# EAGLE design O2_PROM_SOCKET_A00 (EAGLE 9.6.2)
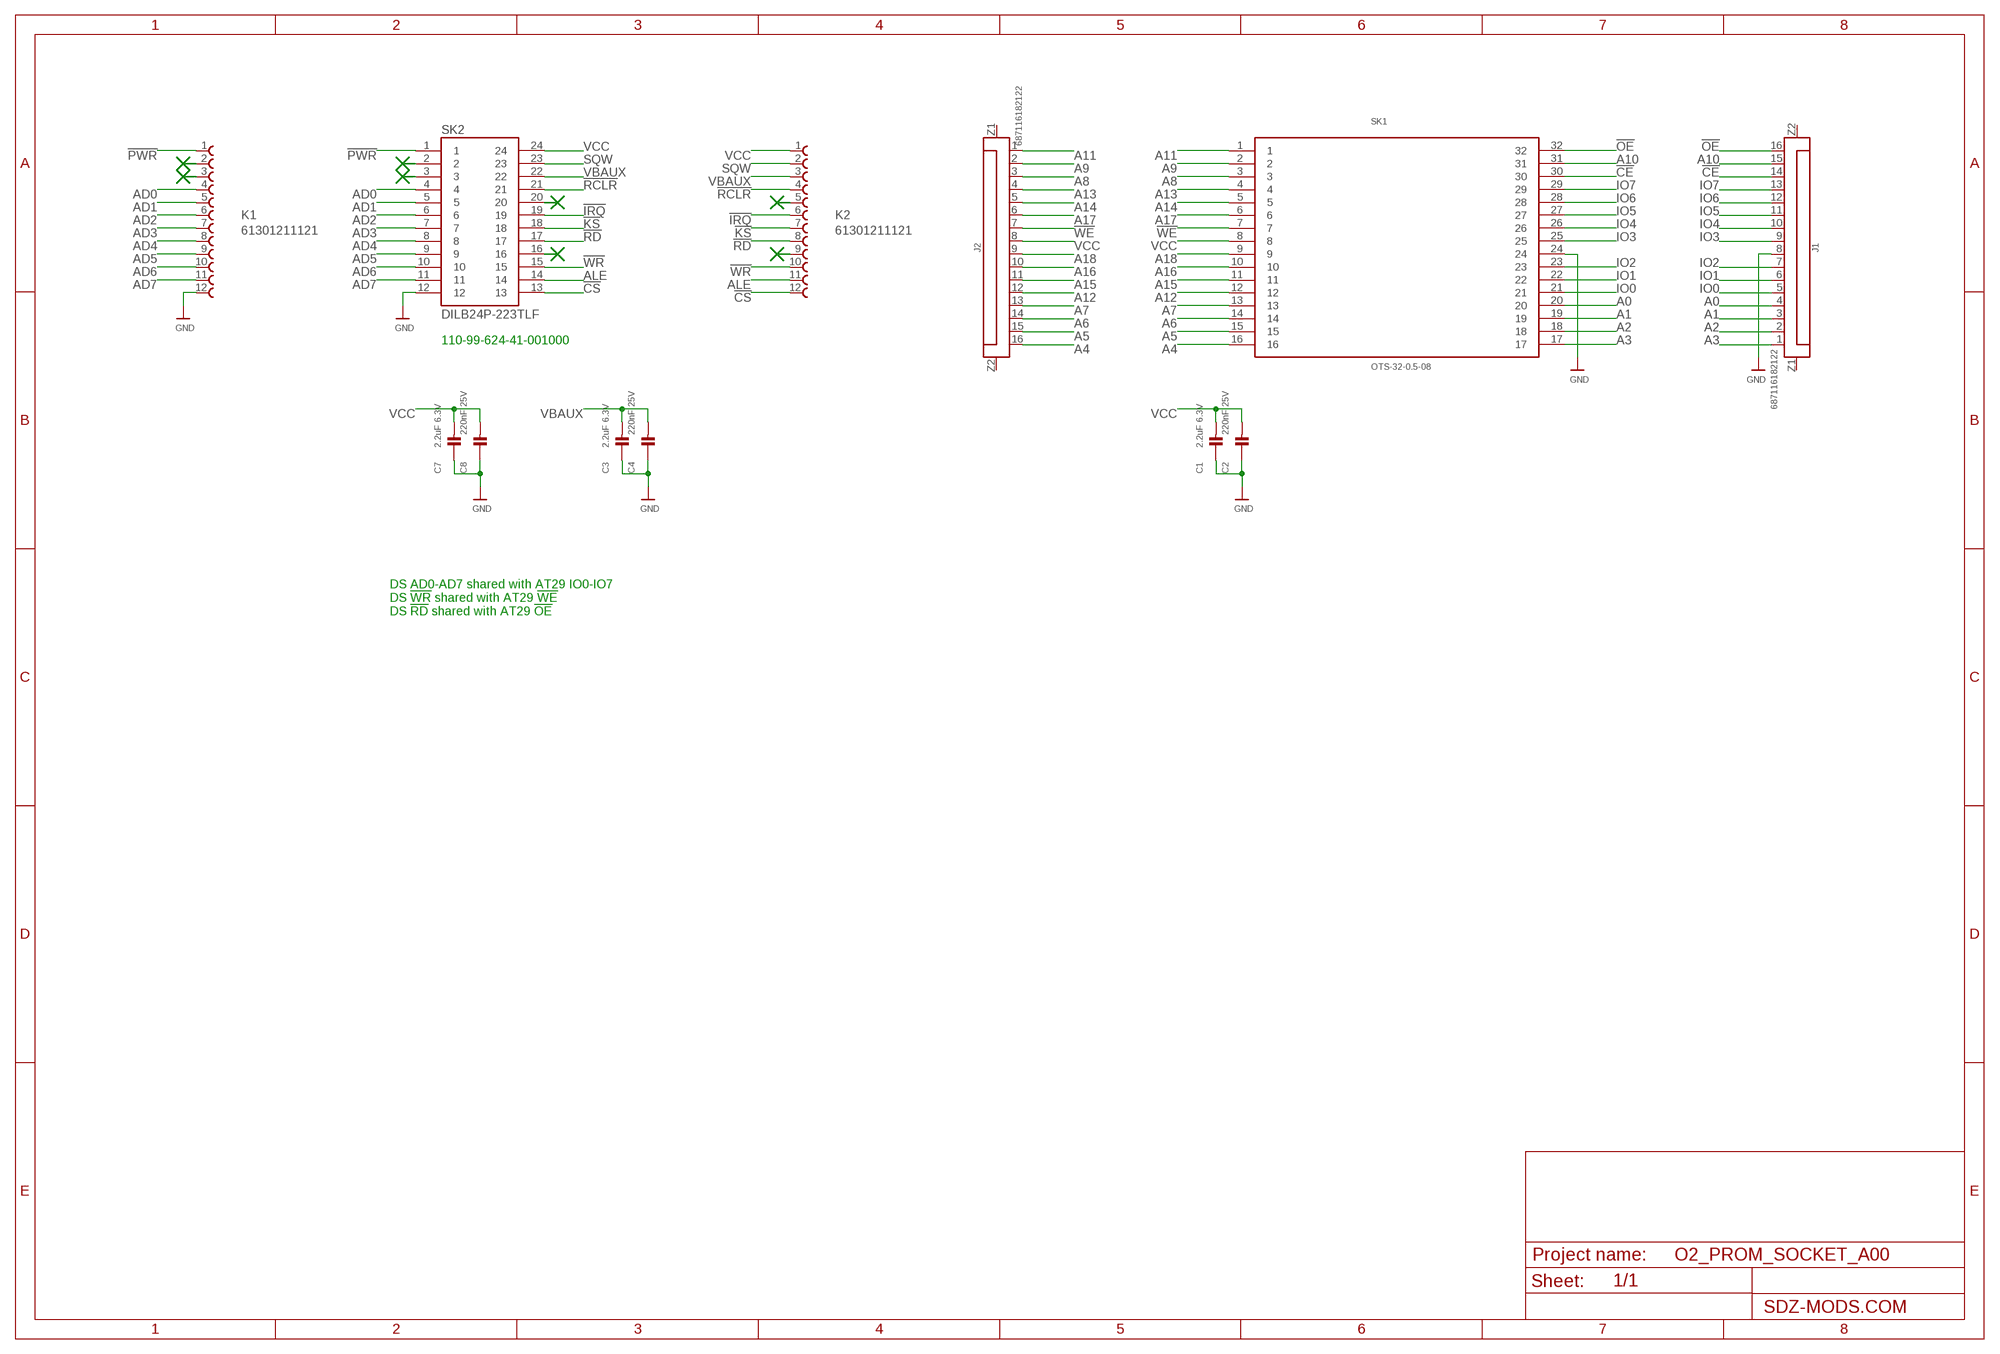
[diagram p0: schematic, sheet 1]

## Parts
C1  2.2uF 6.3V  CAP_CERAMIC0402D  [0402D]
C2  220nF 25V  CAP_CERAMIC0402D  [0402D]
C3  2.2uF 6.3V  CAP_CERAMIC0402D  [0402D]
C4  220nF 25V  CAP_CERAMIC0402D  [0402D]
C7  2.2uF 6.3V  CAP_CERAMIC0402D  [0402D]
C8  220nF 25V  CAP_CERAMIC0402D  [0402D]
J1  687116182122  6871XX182122_687116182122  [687116182122]
J2  687116182122  6871XX182122_687116182122  [687116182122]
K1  61301211121  [61301211121]
K2  61301211121  [61301211121]
SK1  OTS-32-0.5-08  [OTS-32-0.5-08]
SK2  DILB24P-223TLF  [AMPHENOL_DILB24P-223TLF]

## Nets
!CE: J1.14 SK1.30
!CS: K2.12 SK2.13
!IRQ: K2.6 SK2.19
!KS: K2.7 SK2.18
!OE: J1.16 SK1.32
!PWR: K1.1 SK2.1
!RCLR: K2.4 SK2.21
!RD: K2.8 SK2.17
!WE: J2.7 SK1.7
!WR: K2.10 SK2.15
A0: J1.4 SK1.20
A1: J1.3 SK1.19
A2: J1.2 SK1.18
A3: J1.1 SK1.17
A4: J2.16 SK1.16
A5: J2.15 SK1.15
A6: J2.14 SK1.14
A7: J2.13 SK1.13
A8: J2.3 SK1.3
A9: J2.2 SK1.2
A10: J1.15 SK1.31
A11: J2.1 SK1.1
A12: J2.12 SK1.12
A13: J2.4 SK1.4
A14: J2.5 SK1.5
A15: J2.11 SK1.11
A16: J2.10 SK1.10
A17: J2.6 SK1.6
A18: J2.9 SK1.9
AD0: K1.4 SK2.4
AD1: K1.5 SK2.5
AD2: K1.6 SK2.6
AD3: K1.7 SK2.7
AD4: K1.8 SK2.8
AD5: K1.9 SK2.9
AD6: K1.10 SK2.10
AD7: K1.11 SK2.11
ALE: K2.11 SK2.14
GND: C1.3 C2.3 C3.3 C4.3 C7.3 C8.3 J1.8 K1.12 SK1.24 SK2.12
IO0: J1.5 SK1.21
IO1: J1.6 SK1.22
IO2: J1.7 SK1.23
IO3: J1.9 SK1.25
IO4: J1.10 SK1.26
IO5: J1.11 SK1.27
IO6: J1.12 SK1.28
IO7: J1.13 SK1.29
SQW: K2.2 SK2.23
VBAUX: C3.4 C4.4 K2.3 SK2.22
VCC: C1.4 C2.4 C7.4 C8.4 J2.8 K2.1 SK1.8 SK2.24
Unconnected: J1.Z1 J1.Z2 J2.Z1 J2.Z2 K1.2 K1.3 K2.5 K2.9 SK2.2 SK2.3 SK2.16 SK2.20

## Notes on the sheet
- 110-99-624-41-001000
- DS AD0-AD7 shared with AT29 IO0-IO7
  DS !WR! shared with AT29 !WE!
  DS !RD! shared with AT29 !OE!

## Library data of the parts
C1-C4 C7 C8 = microbuilder:CAP_CERAMIC: Ceramic Capacitors
J1 J2 = Eagle_WR-FPC (rev24a):6871XX182122_687116182122: WR-FPC 0.50 mm SMT ZIF Horizontal Dual Contact KIND PROPERTIES Pitch 0.5 mm MATERIAL PROPERTIES Insulator Material LCP Contact Material Phosphor Bronze Contact Plating 80 (µ") Tin over 50 (µ") Nickel Contact Type Stamped Solder Tabs Brass Details see: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; CONTACT-RESISTANCE: 30mOhm; DATASHEET-URL: https://www.we-online.com/redexpert/spec/687116182122?ae; IR: 0.5A; L: 10mm; PACKAGING: Tape and Reel; PART-NUMBER: 687116182122; PINS: 16; PITCH: 0.5mm; TYPE: Horizontal; WORKING-VOLTAGE: 50V(AC)
K1 K2 = Wuerth_Elektronik_eiCan_Board_to_Board_Connectors:61301211121: WR-PHD 2.54mm Pin Header, 12 Pins =>Code : Con_BTB_PHD_2.54_1_THT_61301211121 Details see: http://katalog.we-online.de/en/em/613_0xx_111_21 Created 2014-05-29, Karrer Zheng 2014 (C) Würth Elektronik
SK1 = OTS-32-0_5-08:OTS-32-0.5-08
SK2 = DILB24P-223TLF:DILB24P-223TLF

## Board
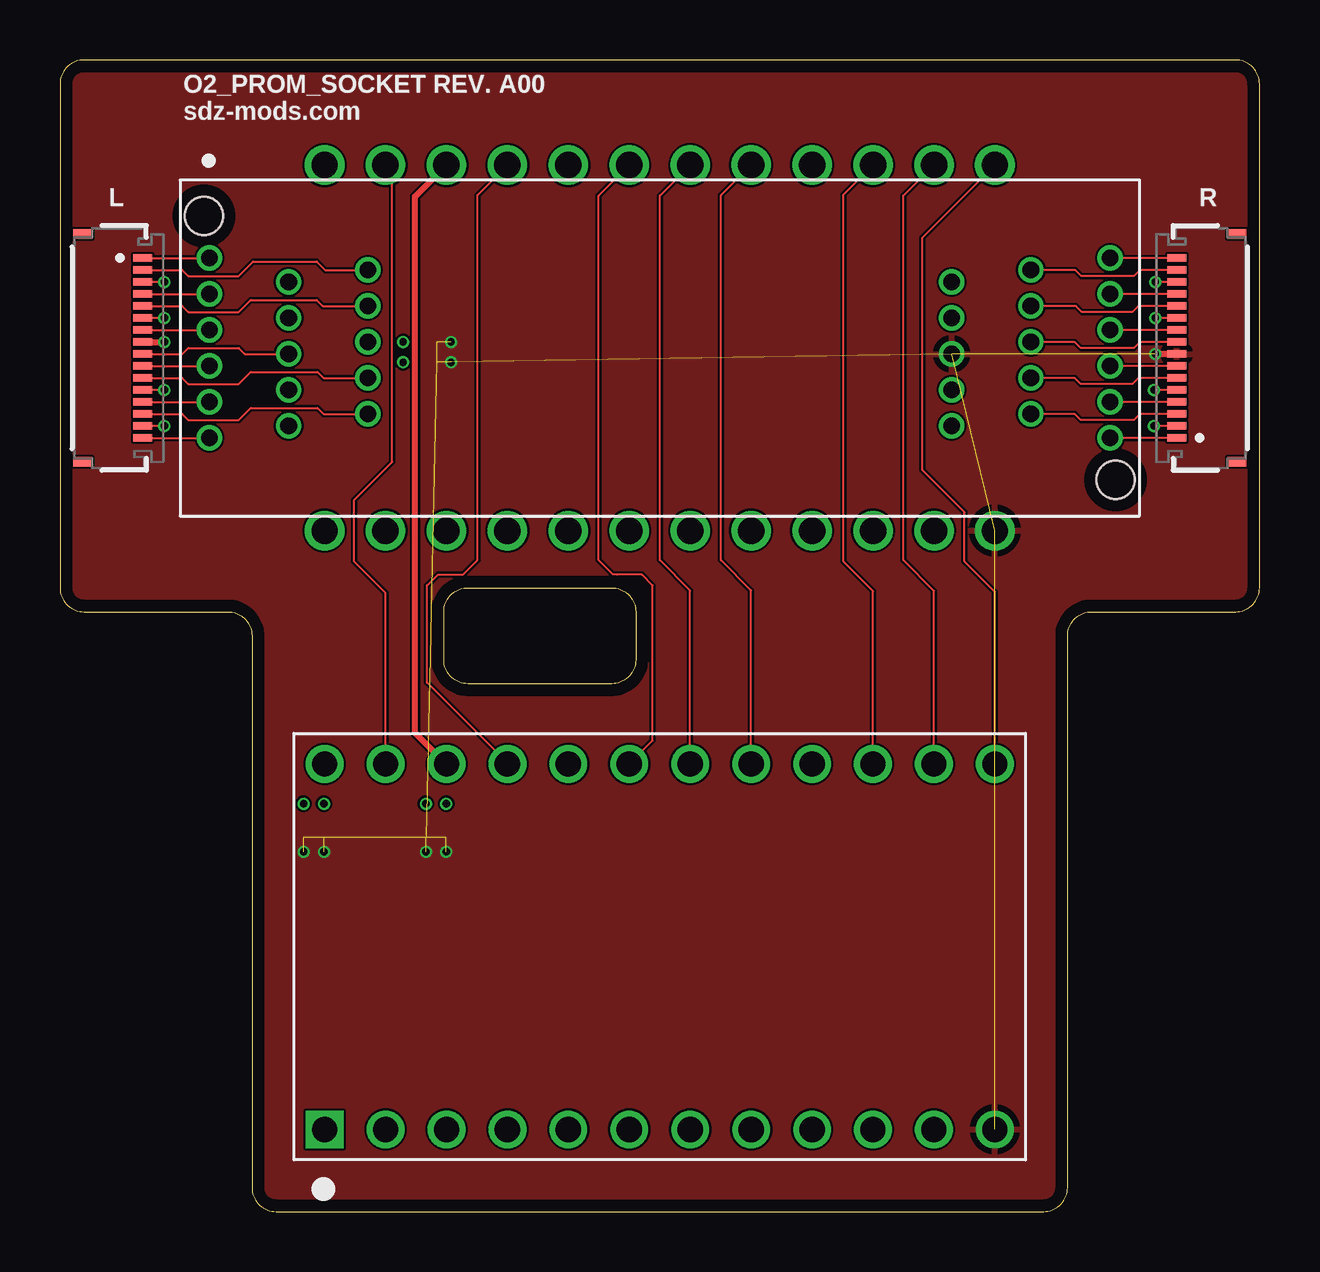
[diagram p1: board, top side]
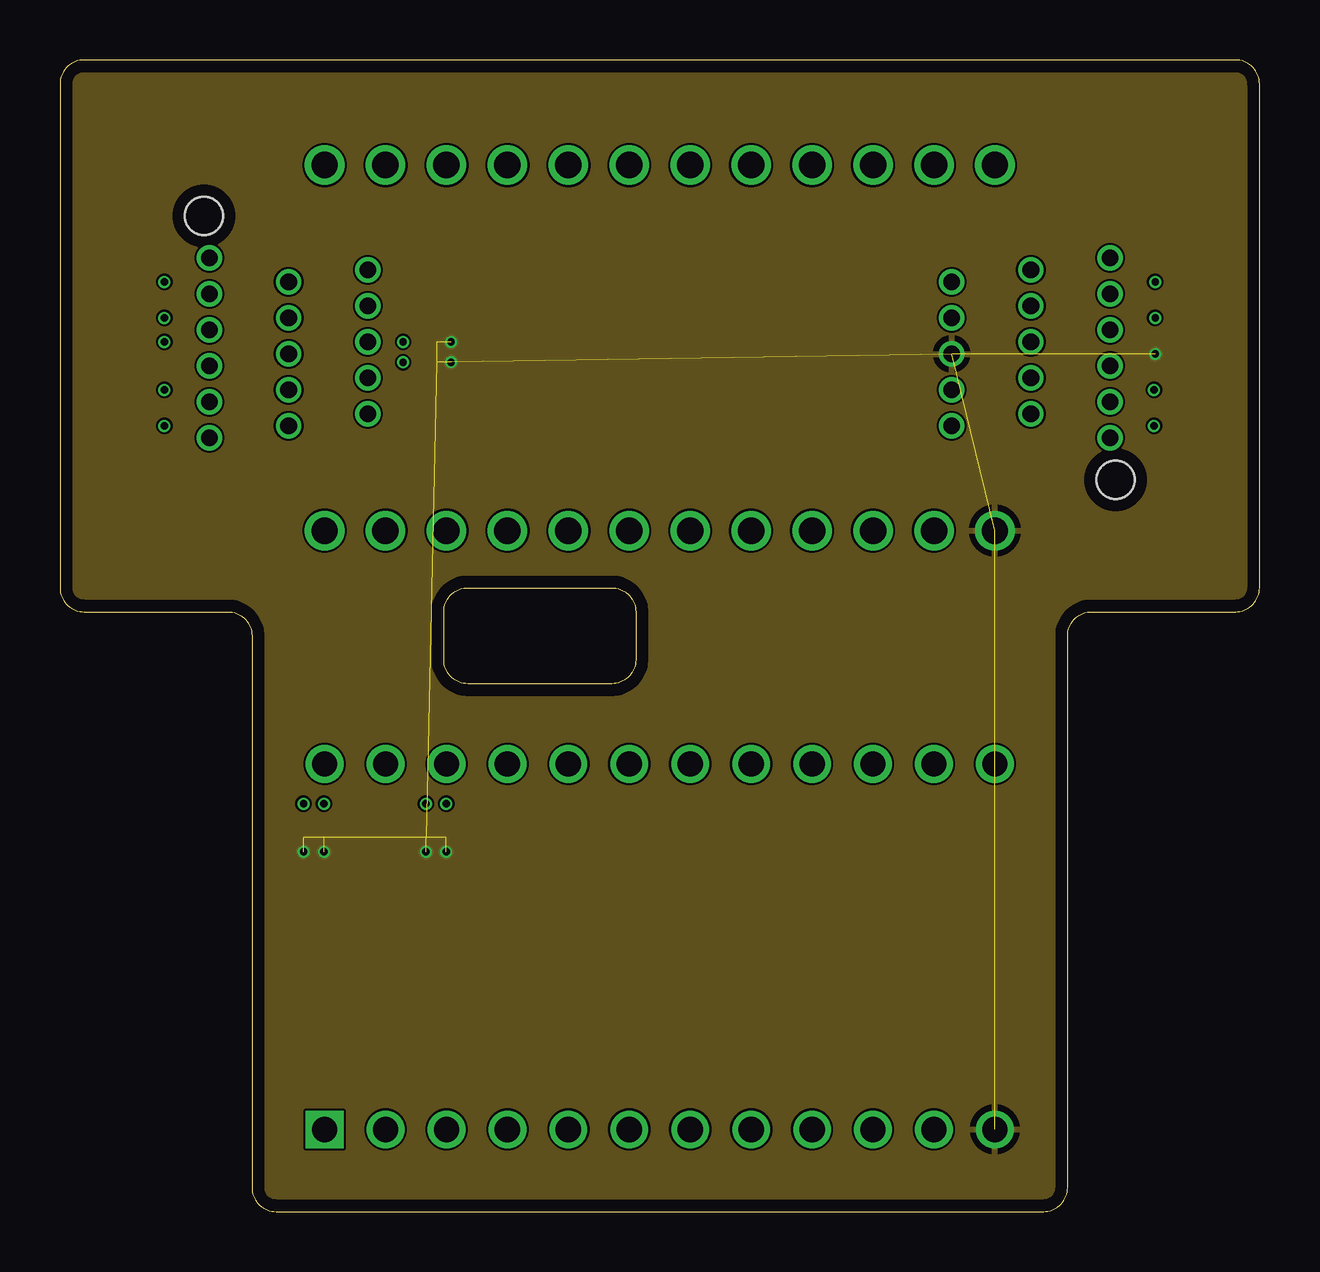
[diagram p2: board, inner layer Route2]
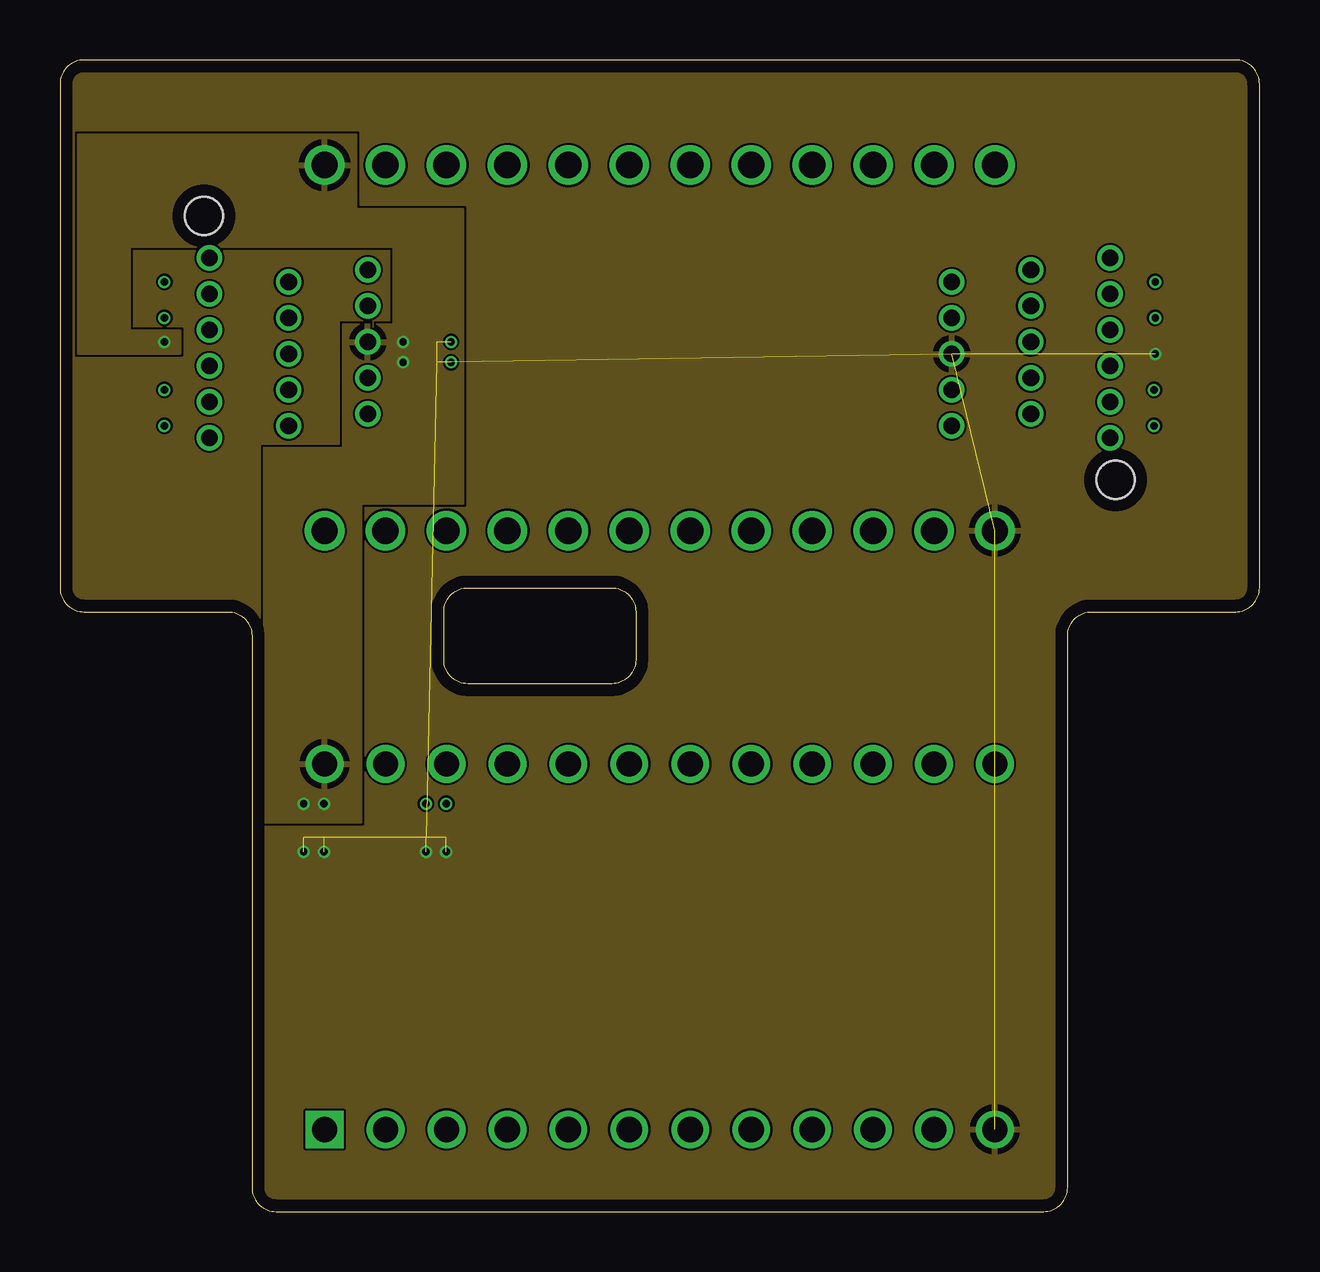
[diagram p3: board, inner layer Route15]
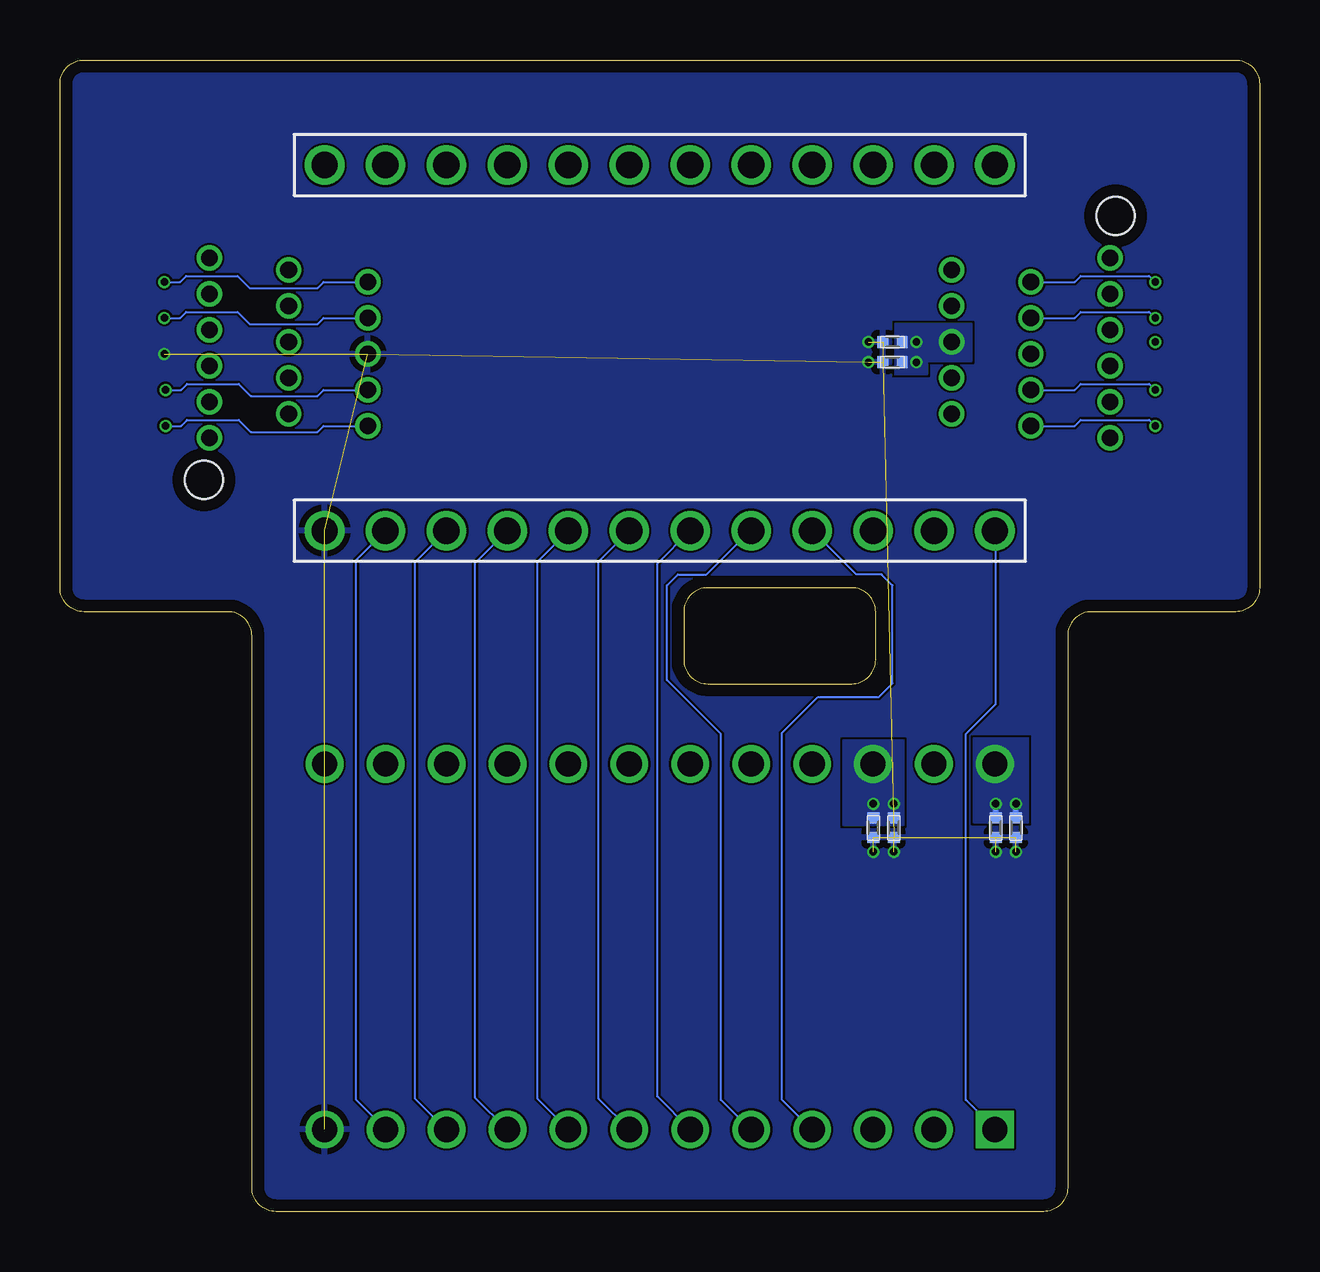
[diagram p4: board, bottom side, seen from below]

Size 50 x 48 mm. Coordinates in mm from the lower left corner, seen from the top.
Outline: 0,47 0,26 arc90 1,25 7,25 arc-90 8,24 8,1 arc90 9,0 41,0 arc90 42,1 42,24 arc-90 43,25 49,25 arc90 50,26 50,47 arc90 49,48 1,48 arc90 0,47
Outline: 17,26 23,26 arc-90 24,25 24,23 arc-90 23,22 17,22 arc-90 16,23 16,25 arc-90 17,26
Copper layers (1+2*15+16): Top 0.035mm / dielectric 1.5mm / Route2 0.035mm / dielectric 0.15mm / Route15 0.035mm / dielectric 0.2mm / Bottom 0.035mm
Design rules "default *": minimum track width 0.09mm, minimum drill 0.3mm, track to track 0.09mm, track to pad 0.09mm, pad to pad 0.09mm, via to via 0.09mm, smd to smd 0.09mm, copper to edge 20mil, drill to drill 6mil, minimum pad ring 7mil, minimum via ring 0.1mm, stop-mask expansion 4mil, vias tented up to drill 0.35mm, thermal gap 10mil

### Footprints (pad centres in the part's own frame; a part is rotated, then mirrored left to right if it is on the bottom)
0402D = smd 0.45 x 0.5: 3 -0.403,0; 4 0.404,0
687116182122 = smd 0.3 x 0.8: 1 -3.75,1.4; 2 -3.25,1.4; 3 -2.75,1.4; 4 -2.25,1.4; 5 -1.75,1.4; 6 -1.25,1.4; 7 -0.75,1.4; 8 -0.25,1.4; 9 0.25,1.4; 10 0.75,1.4; 11 1.25,1.4; 12 1.75,1.4; 13 2.25,1.4; 14 2.75,1.4; 15 3.25,1.4; 16 3.75,1.4 | smd 0.4 x 0.8: Z1 -4.75,-1.1; Z2 4.75,-1.1
61301211121 = drill 1.1: 1 -13.97,0; 2 -11.43,0; 3 -8.89,0; 4 -6.35,0; 5 -3.81,0; 6 -1.27,0; 7 1.27,0; 8 3.81,0; 9 6.35,0; 10 8.89,0; 11 11.43,0; 12 13.97,0
OTS-32-0.5-08 = drill 0.7: 1 -18.77,3.75; 2 -12.17,3.25; 3 -15.47,2.75; 4 -18.77,2.25; 5 -12.17,1.75; 6 -15.47,1.25; 7 -18.77,0.75; 8 -12.17,0.25; 9 -15.47,-0.25; 10 -18.77,-0.75; 11 -12.17,-1.25; 12 -15.47,-1.75; 13 -18.77,-2.25; 14 -12.17,-2.75; 15 -15.47,-3.25; 16 -18.77,-3.75; 17 18.77,-3.75; 18 12.17,-3.25; 19 15.47,-2.75; 20 18.77,-2.25; 21 12.17,-1.75; 22 15.47,-1.25; 23 18.77,-0.75; 24 12.17,-0.25; 25 15.47,0.25; 26 18.77,0.75; 27 12.17,1.25; 28 15.47,1.75; 29 18.77,2.25; 30 12.17,2.75; 31 15.47,3.25; 32 18.77,3.75 | hole 1.6: 19,-5.5; -19,5.5
AMPHENOL_DILB24P-223TLF = drill 1.05 square: 1 -7.62,13.97 | drill 1.05: 2 -7.62,11.43; 3 -7.62,8.89; 4 -7.62,6.35; 5 -7.62,3.81; 6 -7.62,1.27; 7 -7.62,-1.27; 8 -7.62,-3.81; 9 -7.62,-6.35; 10 -7.62,-8.89; 11 -7.62,-11.43; 12 -7.62,-13.97; 13 7.62,-13.97; 14 7.62,-11.43; 15 7.62,-8.89; 16 7.62,-6.35; 17 7.62,-3.81; 18 7.62,-1.27; 19 7.62,1.27; 20 7.62,3.81; 21 7.62,6.35; 22 7.62,8.89; 23 7.62,11.43; 24 7.62,13.97

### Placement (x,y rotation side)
C1  15.3,35.4 0 bottom
C2  15.3,36.25 0 bottom
C3  15.25,16 90 bottom
C4  16.1,16 90 bottom
C7  10.15,16 90 bottom
C8  11,16 90 bottom
J1  47.95,36 90 top
J2  2.05,36 270 top
K1  25,28.38 180 bottom
K2  25,43.62 180 bottom
SK1  25,36 0 top
SK2  25,11.04 90 top

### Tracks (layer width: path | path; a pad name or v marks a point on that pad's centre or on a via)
!CE  (via drill 0.3)
  Top 0.09: J1.14 v45.65,38.75
  Bottom 0.09: v45.65,38.75 45,38.75 44.75,39 42.6,39 42.1,38.5 39.27,38.5 39.02,38.75 SK1.30
!CS
  Top 0.09: SK2.13 38.97,25.83 37.7,27.1 37.7,29.15 35.95,30.9 35.95,40.6 K2.12
!IRQ
  Top 0.09: SK2.19 24.7,19.63 24.7,26.1 24.25,26.55 23.23,26.55 23.05,26.55 22.45,27.15 22.45,42.34 K2.6
!KS
  Top 0.09: SK2.18 26.27,25.88 25,27.15 25,42.35 K2.7
!OE
  Top 0.09: J1.16 SK1.32
!PWR
  Bottom 0.09: SK2.1 12.25,4.65 12.25,19.9 11,21.15 11,28.35 K1.1
!RCLR
  Top 0.09: SK2.21 18.65,18.7 15.3,22.05 15.3,26.1 15.75,26.55 16.8,26.55 17.4,27.15 17.4,42.37 K2.4
!RD
  Top 0.09: SK2.17 28.81,25.89 27.55,27.15 27.55,42.36 K2.8
!WE
  Top 0.09: J2.7 SK1.7
!WR
  Top 0.09: SK2.15 33.89,25.86 32.65,27.1 32.65,42.38 K2.10
A0
  Top 0.09: J1.4 SK1.20
A1
  Top 0.09: J1.3 45,33.25 44.75,33 42.55,33 42.3,33.25 SK1.19
A2  (via drill 0.3)
  Top 0.09: J1.2 v45.6,32.75
  Bottom 0.09: v45.6,32.75 44.95,32.75 44.7,33 42.55,33 42.05,32.5 39.27,32.5 39.02,32.75 SK1.18
A3
  Top 0.09: J1.1 SK1.17
A4
  Top 0.09: J2.16 SK1.16
A5  (via drill 0.3)
  Top 0.09: v4.35,32.75 J2.15
  Bottom 0.09: SK1.15 7.7,32.75 7.45,33 4.6,33 v4.35,32.75
A6
  Top 0.09: J2.14 5.1,33.25 5.35,33 7.45,33 7.95,33.5 10.73,33.5 10.98,33.25 SK1.14
A7
  Top 0.09: J2.13 SK1.13
A8  (via drill 0.3)
  Top 0.09: v4.35,38.75 J2.3
  Bottom 0.09: SK1.3 7.7,38.75 7.45,39 4.6,39 v4.35,38.75
A9
  Top 0.09: J2.2 5.1,39.25 5.35,39 7.45,39 8.05,39.6 10.7,39.6 11.05,39.25 SK1.2
A10
  Top 0.09: J1.15 45,39.25 44.75,39 42.57,39 42.32,39.25 SK1.31
A11
  Top 0.09: J2.1 SK1.1
A12  (via drill 0.3)
  Top 0.09: v4.35,34.25 J2.12
  Bottom 0.09: SK1.12 7.7,34.25 7.45,34.5 4.6,34.5 v4.35,34.25
A13
  Top 0.09: J2.4 SK1.4
A14
  Top 0.09: J2.5 5.1,37.75 5.35,37.5 7.45,37.5 7.95,38 10.7,38 10.95,37.75 SK1.5
A15
  Top 0.09: J2.11 5.1,34.75 5.35,34.5 7.45,34.5 7.95,35 10.73,35 10.98,34.75 SK1.11
A16
  Top 0.09: J2.10 SK1.10
A17  (via drill 0.3)
  Top 0.09: v4.35,37.25 J2.6
  Bottom 0.09: SK1.6 7.7,37.25 7.45,37.5 4.6,37.5 v4.35,37.25
A18
  Top 0.09: J2.9 5.1,35.75 5.35,36 7.45,36 7.7,35.75 SK1.9
AD0
  Bottom 0.09: SK2.4 18.67,3.42 19.9,4.65 19.9,19.95 18.4,21.45 15.87,21.45 15.3,22.02 15.3,26.1 15.75,26.55 16.8,26.55 18.63,28.38 K1.4
AD1
  Bottom 0.09: K1.5 21.22,28.38 23.05,26.55 24.25,26.55 24.7,26.1 24.7,22.15 22.45,19.9 22.45,4.65 21.22,3.42 SK2.5
AD2
  Bottom 0.09: SK2.6 25.1,4.8 25.1,27.01 K1.6
AD3
  Bottom 0.09: K1.7 27.55,27.1 27.55,4.7 SK2.7
AD4
  Bottom 0.09: K1.8 30.1,27.09 30.1,4.7 SK2.8
AD5
  Bottom 0.09: K1.9 32.7,27.03 32.7,4.75 31.37,3.42 SK2.9
AD6
  Bottom 0.09: K1.10 35.2,27.07 35.2,4.7 33.92,3.42 SK2.10
AD7
  Bottom 0.09: SK2.11 37.65,4.65 37.65,27.16 K1.11
ALE
  Top 0.09: SK2.14 36.43,25.87 35.15,27.15 35.15,42.35 K2.11
GND  (via drill 0.3)  (15 unrouted)
  Top 0.254: J1.8 v45.65,35.75
  other vias: 11,15 10.15,15 16.3,36.25 16.3,35.4 15.25,15 16.1,15
  pour Top (rank 5): -1.5,49.9 51.85,49.9 51.85,-1.95 -1.5,-1.95
  pour Route2 (rank 5): -1.5,49.9 51.85,49.9 51.85,-1.95 -1.5,-1.95
  pour Route15 (rank 5): -1.5,49.9 51.85,49.9 51.85,-1.95 -1.5,-1.95
  pour Bottom (rank 5): -1.5,49.9 51.85,49.9 51.85,-1.95 -1.5,-1.95
IO0  (via drill 0.3)
  Top 0.09: J1.5 v45.6,34.25
  Bottom 0.09: v45.6,34.25 44.95,34.25 44.7,34.5 42.55,34.5 42.05,34 39.27,34 39.02,34.25 SK1.21
IO1
  Top 0.09: J1.6 44.95,34.75 44.7,34.5 42.55,34.5 42.3,34.75 SK1.22
IO2
  Top 0.09: J1.7 SK1.23
IO3
  Top 0.09: J1.9 45,36.25 44.75,36 42.55,36 42.3,36.25 SK1.25
IO4
  Top 0.09: J1.10 SK1.26
IO5  (via drill 0.3)
  Top 0.09: J1.11 v45.65,37.25
  Bottom 0.09: v45.65,37.25 45,37.25 44.75,37.5 42.6,37.5 42.1,37 39.27,37 39.02,37.25 SK1.27
IO6
  Top 0.09: J1.12 44.95,37.75 44.7,37.5 42.6,37.5 42.35,37.75 SK1.28
IO7
  Top 0.09: J1.13 SK1.29
SQW
  Top 0.09: SK2.23 13.57,25.78 12.25,27.1 12.25,29.65 13.85,31.25 13.85,43.34 K2.2
VBAUX  (via drill 0.3)
  Top 0.09: SK2.22 16.09,18.66
  Top 0.254: K2.3 14.8,42.31 14.8,19.95 16.09,18.66
  other vias: 16.1,17 15.25,17
  pour Bottom (no thermals): 14.85,16.1 17.35,16.1 17.35,19.65 14.85,19.65
VCC  (via drill 0.3)
  Top 0.254: J2.8 v4.35,36.25
  Bottom 0.254: C8.4 v11,17 | C7.4 v10.15,17
  other vias: 14.3,36.25 14.3,35.4
  pour Route15: 0.75,44.9 12.35,44.9 12.35,41.8 16.8,41.8 16.8,29.5 12.55,29.5 12.55,16.2 8.5,16.2 8.5,31.85 11.8,31.85 11.8,37 13.9,37 13.9,40.2 2.9,40.2 2.9,36.75 5,36.75 5,35.75 0.75,35.75
  pour Bottom (no thermals): 9.65,16.2 11.9,16.2 11.9,19.75 9.65,19.75
  pour Bottom (no thermals): 12,37 15.2,37 15.2,34.9 13.85,34.9 13.85,35.45 12,35.45

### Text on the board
tPlace: O2_PROM_SOCKET REV. A00 / sdz-mods.com | L | R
